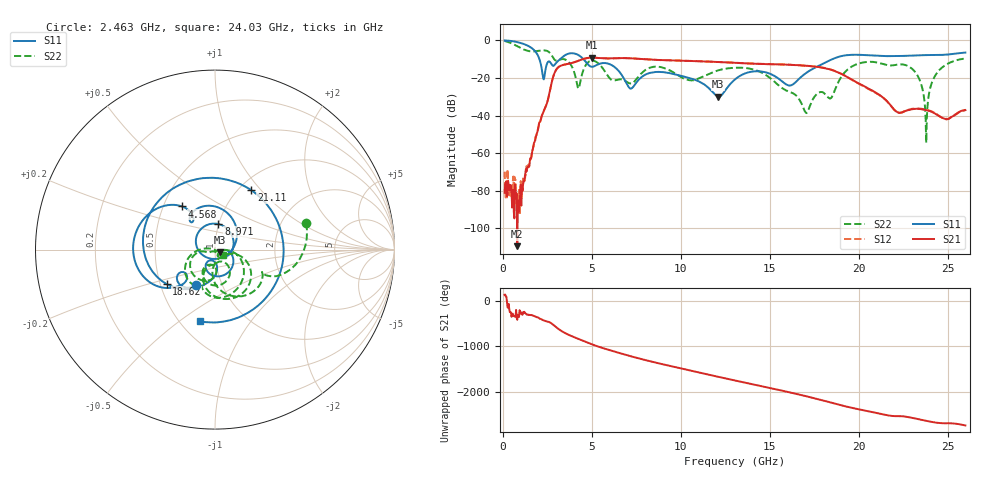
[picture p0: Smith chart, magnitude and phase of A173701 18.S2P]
!  2-Port S-parameters saved by WinCal
! VAR MeasName=S-Parameters (CALIBRATED_DATA) read from VNA (N5245A)
! VAR MeasDate=2017-6-7 10:29:34
! VAR NAME=A173701 18
! VAR FILENAME=A173701 18.S2P
! VAR DATE=2017-6-7 10:29:34
! VAR PHYS_PORTS=1,2
# Hz S DB R 50
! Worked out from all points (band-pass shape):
!   801 points, 100 MHz to 26 GHz, reference 50 ohm
!   highest |S21| = -9.15 dB at 5.021 GHz (marker M1); lowest = -109.6 dB at 812.2 MHz (marker M2)
!   |S21| within 3 dB of the highest: 3.826 GHz to 13.56 GHz (9.736 GHz wide, 112 % of centre)
!   lowest |S11| = -30.0 dB at 12.11 GHz (marker M3), VSWR 1.07, Z = 52.9 - j1.54 ohm
!   |S11| at or under -10 dB: 2.058 GHz to 3.215 GHz (1.158 GHz wide, 43.9 % of centre); 4.531 GHz to 18.52 GHz (13.99 GHz wide, 121 % of centre)
!   |S22| runs from -54.5 to -0.2 dB; largest |S21 - S12| = 0.0038
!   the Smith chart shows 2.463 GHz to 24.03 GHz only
!   S11 on the Smith chart (normalised r, x): 2.463 GHz: 0.75, -0.32; 4.568 GHz: 0.62, +0.33; 8.971 GHz: 1.00, +0.29; 18.62 GHz: 0.54, -0.23; 21.11 GHz: 1.14, +0.89; 24.03 GHz: 0.63, -0.60
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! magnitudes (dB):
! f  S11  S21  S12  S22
! 100 MHz  0.0  -81.2  -69.9  -0.2
! 812.2 MHz  -0.9  -109.6  -85.2  -3.1
! 2.463 GHz  -12.9  -33.9  -33.9  -5.5
! 3.046 GHz  -11.5  -15.0  -15.0  -10.7
! 4.438 GHz  -9.1  -10.1  -10.2  -18.5
! 4.568 GHz  -10.4  -9.8  -9.8  -14.9
! 5.021 GHz  -14.0  -9.1  -9.2  -10.8
! 7.158 GHz  -25.6  -9.5  -9.5  -22.9
! 8.744 GHz  -16.7  -10.4  -10.4  -14.0
! 8.971 GHz  -16.9  -10.5  -10.5  -14.4
! 12.11 GHz  -30.0  -11.5  -11.5  -15.9
! 13.05 GHz  -20.8  -11.9  -11.9  -14.6
! 16.16 GHz  -24.0  -13.0  -13.0  -27.6
! 17.39 GHz  -15.3  -13.8  -13.7  -32.1
! 18.62 GHz  -9.6  -16.2  -16.1  -27.5
! 19.56 GHz  -7.7  -20.5  -20.6  -14.3
! 21.11 GHz  -8.2  -28.7  -28.8  -11.9
! 21.69 GHz  -8.4  -33.4  -33.5  -13.3
! 23.15 GHz  -8.0  -36.5  -36.3  -16.5
! 23.8 GHz  -7.8  -37.1  -36.9  -54.5
! 24.03 GHz  -7.8  -37.8  -37.5  -25.3
! 26 GHz  -6.5  -37.1  -37.0  -9.7
